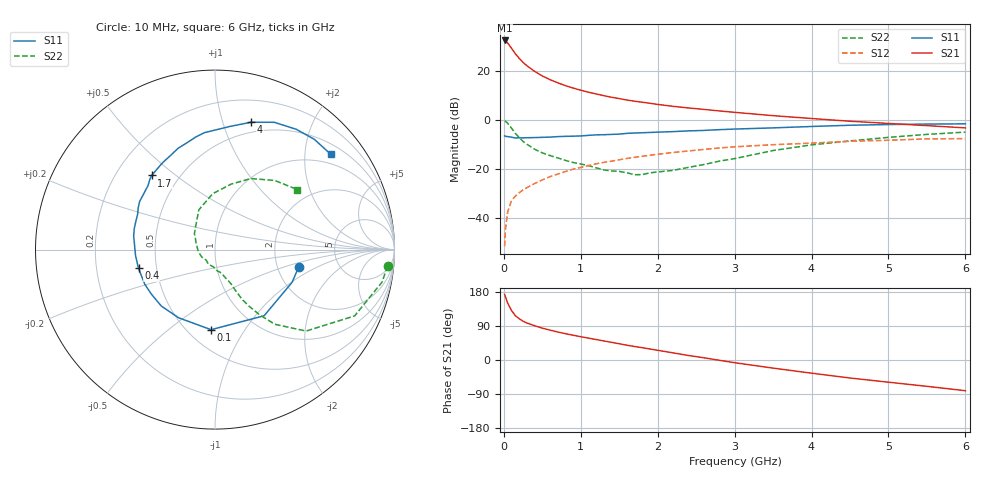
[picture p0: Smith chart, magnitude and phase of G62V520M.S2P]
! SIEMENS Small Signal Semiconductors
! BFG193
! Si NPN RF Bipolar Junction Transistor in SOT223
! VCE = 2.5 V  IC = 20 mA
! Common Emitter S-Parameters:  August  1996
# GHz  S  MA  R  50
!  f  S11  S21  S12  S22
! GHz  MAG  ANG  MAG  ANG  MAG  ANG  MAG  ANG
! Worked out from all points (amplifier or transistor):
!   36 points, 10 MHz to 6 GHz, reference 50 ohm
!   highest |S21| = 32.4 dB at 10 MHz (marker M1)
!   |S21| within 3 dB of that: start of sweep to 95.69 MHz
!   unconditionally stable (mu >= 1): 671.5 MHz to 2.603 GHz
!   at 250 MHz: K = 0.75, MSG = 26.0 dB, |S12| = -28.5 dB
!   at 1.4 GHz: K = 1.06, MAG = 11.5 dB, |S12| = -16.8 dB
!   at 6 GHz: K = 0.90, MSG = 2.2 dB, |S12| = -7.6 dB
!   S11 on the Smith chart (normalised r, x): 10 MHz: 2.63, -0.66; 100 MHz: 0.64, -0.72; 400 MHz: 0.39, -0.10; 1.7 GHz: 0.35, +0.41; 4 GHz: 0.40, +1.24; 6 GHz: 0.74, +2.60
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0.01  0.4762 -11.7  41.66 173.2  0.0027 87.7  0.9656 -5.4
0.02  0.4668 -22.9  40.91 167.6  0.0058 81.7  0.9483 -11.0
0.05  0.4591 -53.4  36.9 149.8  0.0135 72.2  0.8611 -25.4
0.1  0.4467 -92.8  28.88 130.6  0.0229 62.7  0.6808 -41.8
0.15  0.4306 -118.1  22.26 116.9  0.0282 57.5  0.5333 -51.3
0.2  0.4341 -133.6  18.03 108.9  0.0331 57.6  0.4393 -55.7
0.25  0.4329 -145.4  14.92 102.4  0.0378 57.2  0.3665 -59.0
0.3  0.4361 -153.9  12.72 97.6  0.0419 58.3  0.321 -61.2
0.4  0.4388 -166.2  9.784 90.5  0.0509 59.3  0.2544 -63.4
0.5  0.444 -175.8  7.887 84.0  0.0603 59.4  0.2142 -64.7
0.6  0.4485 177.1  6.644 78.9  0.0703 59.9  0.189 -66.7
0.7  0.4593 170.6  5.728 73.9  0.0791 59.3  0.1694 -69.5
0.9  0.4687 159.8  4.476 65.4  0.0998 56.9  0.1366 -74.4
1.1  0.487 151.4  3.682 57.7  0.1179 54.3  0.118 -84.7
1.4  0.5091 139.4  2.902 46.6  0.1452 48.9  0.0918 -103.6
1.7  0.5432 130.5  2.415 35.6  0.1742 43.2  0.0768 -128.5
2.2  0.5808 115.0  1.899 18.8  0.2182 32.3  0.0944 -176.3
3.5  0.6916 83.0  1.226 -21.4  0.3144 1.9  0.239 112.2
4  0.738 74.1  1.073 -34.8  0.3384 -7.8  0.3117 92.4
4.5  0.7825 65.0  0.944 -47.5  0.3688 -17.9  0.375 76.3
5.5  0.827 48.0  0.768 -69.5  0.4131 -41.2  0.5094 49.1
6  0.8354 39.5  0.691 -81.0  0.418 -54.5  0.5679 36.1
